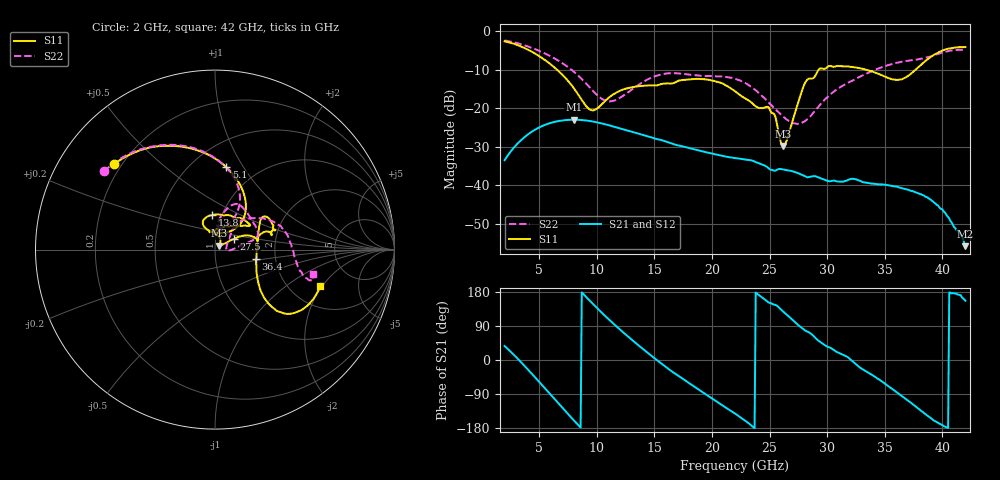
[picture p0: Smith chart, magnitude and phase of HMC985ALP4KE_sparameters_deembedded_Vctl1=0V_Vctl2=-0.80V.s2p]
!s2p File: Measurements: S11, S21, S12, S22
# GHz S dB R 50.0
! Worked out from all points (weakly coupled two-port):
!   401 points, 2 GHz to 42 GHz, reference 50 ohm
!   highest |S21| = -23.01 dB at 8 GHz (marker M1); lowest = -55.9 dB at 42 GHz (marker M2)
!   lowest |S11| = -29.8 dB at 26.2 GHz (marker M3), VSWR 1.07, Z = 52.4 + j2.24 ohm
!   |S11| at or under -10 dB: 6.542 GHz to 29.27 GHz (22.73 GHz wide, 127 % of centre); 33.35 GHz to 37.69 GHz (4.346 GHz wide, 12.2 % of centre)
!   |S22| runs from -24.1 to -2.4 dB; largest |S21 - S12| = 0.00014
!   S11 on the Smith chart (normalised r, x): 2 GHz: 0.17, +0.36; 5.1 GHz: 0.72, +0.84; 13.8 GHz: 0.90, +0.36; 27.5 GHz: 1.22, +0.15; 36.4 GHz: 1.58, -0.17; 42 GHz: 2.90, -1.91
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2  -2.65 140.0  -33.54 36.9  -33.53 36.9  -2.43 144.8
3.5  -4.10 112.1  -28.13 -8.0  -28.14 -8.0  -3.49 120.6
5.1  -6.69 82.1  -24.88 -61.1  -24.88 -61.1  -5.26 96.2
8  -14.79 45.4  -23.01 -159.0  -23.02 -159.0  -10.52 62.3
8.7  -17.89 51.7  -23.10 178.3  -23.11 178.3  -12.46 59.3
9.7  -20.58 86.2  -23.50 147.0  -23.50 146.9  -15.63 61.4
11  -17.39 114.6  -24.41 108.4  -24.41 108.4  -18.24 76.1
13.8  -14.27 95.3  -26.79 34.2  -26.79 34.2  -13.61 77.4
15.4  -13.94 73.0  -28.16 -4.2  -28.16 -4.2  -11.39 68.3
19.4  -12.52 34.6  -31.40 -89.3  -31.40 -89.2  -11.64 35.6
22  -15.59 52.2  -32.98 -141.3  -32.98 -141.3  -12.38 16.3
25  -20.20 97.8  -35.85 150.7  -35.86 150.6  -18.79 4.4
26.2  -29.82 41.5  -35.94 127.3  -35.94 127.3  -22.25 -4.0
27.5  -18.41 29.7  -36.94 91.8  -36.94 91.9  -24.03 4.0
28.1  -13.36 20.7  -37.71 77.7  -37.72 77.7  -23.34 17.3
28.7  -12.32 12.9  -37.74 66.6  -37.70 66.6  -21.59 30.0
31  -9.09 23.4  -39.07 19.0  -39.09 18.8  -14.80 50.3
33.3  -9.96 34.4  -39.37 -28.2  -39.36 -28.4  -11.23 39.5
35.4  -12.27 12.4  -40.08 -71.1  -40.10 -71.2  -8.75 24.5
36.4  -12.57 -12.8  -40.71 -93.3  -40.73 -93.4  -7.97 16.4
39.5  -5.80 -43.2  -45.12 -163.9  -44.95 -163.8  -6.03 -14.7
42  -4.14 -19.0  -55.86 156.2  -56.05 155.7  -4.97 -13.7
